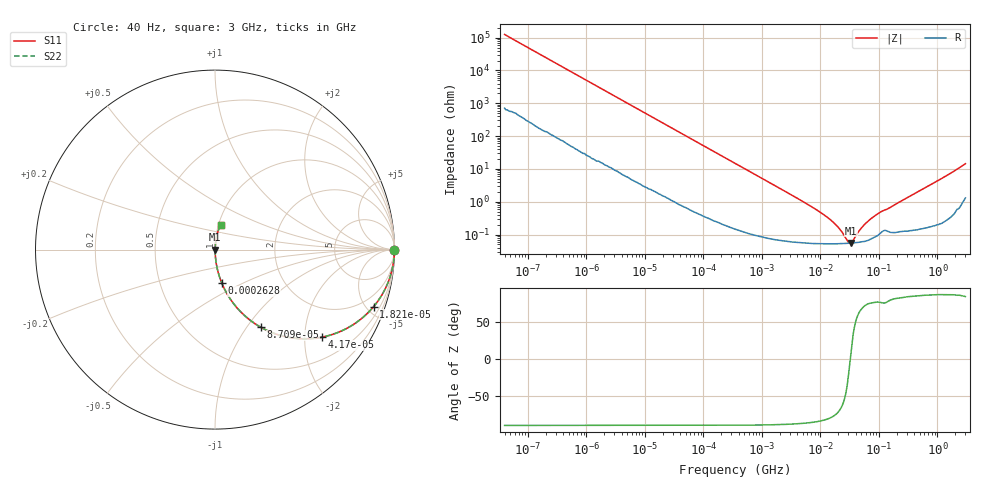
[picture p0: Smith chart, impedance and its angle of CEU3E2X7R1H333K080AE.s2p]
! S-parameter Generated by TDK Corporation
! Copyright(C) 2015 TDK Corporation.
! All Rights Reserved.
! TDK P/N: CEU3E2X7R1H333K080AE (Multilayer Ceramic Chip Capacitors)
! Property: C=33nF
! Size(LxWxT): 1.6x0.8x0.8mm, 0.063x0.031x0.031inches
! Model Type: s2p (Touchstone File Format Version 1.0)
! Frequency: DC=Yes Start=0.00004MHz Stop=3000MHz 396points Log-sweep
! Note: This model was converted from impedance.
! Model Generated on Jun. 23, 2015
! Hash(MD5):
! Port Assignments:
!  1 ---| |--- 2
! Applicable Conditions:
!  Temperature = 25 degC
!  DC Bias Voltage = 0 V
!  Small Signal Operation
! Terms and conditions regarding TDK Simulation Models
! (1)This simulation model is being provided solely for informational purposes. Please refer to the specifications of the products in terms of detailed characteristics of such products.
! (2)In no event shall TDK Corporation of any of its subsidiaries be liable for any loss or damage arising, directly or indirectly,
!  From any information contained in this simulation model, including, but not limited to loss or damages arising from any inaccuracies, omissions or errors in connection with such information.
! (3)Any and all copyrights on this simulation model are owned by TDK Corporation.
!  Duplication or redistribution of this simulation model without prior written permission from TDK Corporation is prohibited.
! (4)This simulation model is subject to any modification or change without any prior notice.
! (5)Neither TDK Corporation nor any of its subsidiaries shall make any warranty, express or implied,
!  Including but not limited to the correctness, implied warranties of merchantability and fitness for a particular purpose with respect to this simulation models.
! (6)The use of this simulation model shall be deemed to have consented to the terms and conditions hereof.
# MHz S MA R 50
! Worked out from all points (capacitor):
!   395 points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, 40 Hz to 3 GHz, reference 50 ohm
!   read as one part in series: C = 32 nF near 41.88 Hz
!   lowest |Z| = 55.2 mohm at 32.99 MHz (marker M1)
!   series resonance near 32.28 MHz, so ESL is about 760 pH
!   S11 on the Smith chart (normalised r, x): 40 Hz: open; 18.21 kHz: 1.03, -5.56; 41.7 kHz: 1.02, -2.44; 87.09 kHz: 1.01, -1.17; 262.8 kHz: 1.00, -0.39; 3 GHz: 1.03, +0.29
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4e-05  1 -0.0  0.0008018 89.6  0.0008018 89.6  1 -0.0
0.000834128  0.9998 -1.0  0.01664 88.7  0.01664 88.7  0.9998 -1.0
0.005020464  0.9945 -5.7  0.09899 84.0  0.09899 84.0  0.9945 -5.7
0.01739424  0.944 -18.9  0.3243 70.7  0.3243 70.7  0.944 -18.9
0.01821348  0.9392 -19.7  0.3378 69.9  0.3378 69.9  0.9392 -19.7
0.04170299  0.7706 -39.2  0.6325 50.4  0.6325 50.4  0.7706 -39.2
0.08708967  0.5035 -59.4  0.8605 30.2  0.8605 30.2  0.5035 -59.4
0.144487  0.3324 -70.2  0.9406 19.4  0.9406 19.4  0.3324 -70.2
0.2628245  0.191 -78.5  0.9799 11.0  0.9799 11.0  0.191 -78.5
0.3464102  0.1463 -81.0  0.9878 8.4  0.9878 8.4  0.1463 -81.0
1.146211  0.04489 -86.4  0.9982 2.6  0.9982 2.6  0.04489 -86.4
7.22376  0.006859 -85.2  0.9994 0.4  0.9994 0.4  0.006859 -85.2
16.54008  0.002376 -77.2  0.9995 0.1  0.9995 0.1  0.002376 -77.2
21.8003  0.001397 -67.6  0.9995 0.1  0.9995 0.1  0.001397 -67.6
30.08671  0.0005857 -22.0  0.9995 0.0  0.9995 0.0  0.0005857 -22.0
32.98752  0.0005515 7.3  0.9995 -0.0  0.9995 -0.0  0.0005515 7.3
47.67047  0.001416 65.4  0.9994 -0.1  0.9994 -0.1  0.001416 65.4
62.83103  0.002409 74.3  0.9994 -0.1  0.9994 -0.1  0.002409 74.3
104.2405  0.004752 76.7  0.9989 -0.3  0.9989 -0.3  0.004752 76.7
150.6385  0.006461 78.9  0.9988 -0.4  0.9988 -0.4  0.006461 78.9
1040.901  0.04481 84.9  0.997 -2.6  0.997 -2.6  0.04481 84.9
3000  0.141 76.7  0.9774 -8.1  0.9774 -8.1  0.141 76.7
